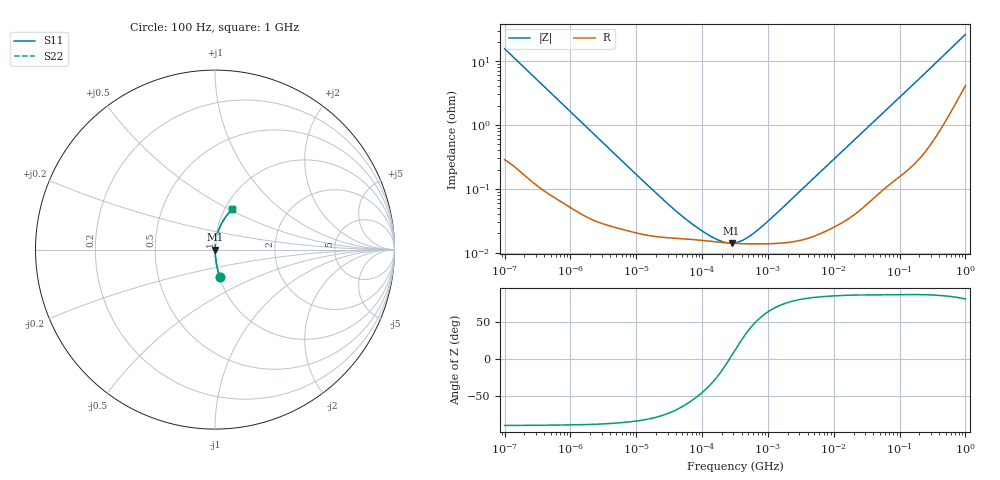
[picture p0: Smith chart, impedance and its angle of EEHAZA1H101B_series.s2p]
!  *** S-Parameter ***
!  Copyright (C) Panasonic Industry
!  Conductive Polymer Hybrid Aluminum Electrolytic Capacitor
!  Parts No. EEHAZA1H101B
!  Connection Mode : Series
!  1  o---||---o  2
!  GND o--------o GND
!  Conditions : Temperature = 20 degC , DC Bias = 0 V
! Frequency Range : 100Hz  -  1GHz  [ 401 Steps ]
# Hz S RI R 50
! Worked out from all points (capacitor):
!   401 points, 100 Hz to 1 GHz, reference 50 ohm
!   read as one part in series: C = 102 uF near 108.4 Hz
!   lowest |Z| = 14.1 mohm at 280.2 kHz (marker M1)
!   series resonance near 259.9 kHz, so ESL is about 3.7 nH
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100  0.0263 -0.151  0.9737 0.151  0.9737 0.151  0.0263 -0.151
108.3927  0.0228 -0.14  0.9772 0.14  0.9772 0.14  0.0228 -0.14
175.7924  0.00968 -0.0882  0.9903 0.0882  0.9903 0.0882  0.00968 -0.0882
309.0295  0.00372 -0.0509  0.9963 0.0509  0.9963 0.0509  0.00372 -0.0509
1487.647  0.000515 -0.0108  0.9995 0.0108  0.9995 0.0108  0.000515 -0.0108
22130.95  0.000177 -0.000758  0.9998 0.000758  0.9998 0.000758  0.000177 -0.000758
51582.22  0.000165 -0.000323  0.9998 0.000323  0.9998 0.000323  0.000165 -0.000323
102329.3  0.000155 -0.00015  0.9998 0.00015  0.9998 0.00015  0.000155 -0.00015
179887.1  0.000146 -5.53e-05  0.9999 5.53e-05  0.9999 5.53e-05  0.000146 -5.53e-05
229086.8  0.000143 -1.89e-05  0.9999 1.89e-05  0.9999 1.89e-05  0.000143 -1.89e-05
280220.6  0.000141 1.14e-05  0.9999 -1.14e-05  0.9999 -1.14e-05  0.000141 1.14e-05
316227.8  0.00014 3e-05  0.9999 -3e-05  0.9999 -3e-05  0.00014 3e-05
454464.5  0.000138 9.05e-05  0.9999 -9.05e-05  0.9999 -9.05e-05  0.000138 9.05e-05
707945.8  0.000137 0.000182  0.9999 -0.000182  0.9999 -0.000182  0.000137 0.000182
1295687  0.00014 0.000371  0.9999 -0.000371  0.9999 -0.000371  0.00014 0.000371
4704354  0.000179 0.00138  0.9998 -0.00138  0.9998 -0.00138  0.000179 0.00138
6.99842e7  0.00152 0.019  0.9985 -0.019  0.9985 -0.019  0.00152 0.019
1.566751e8  0.00399 0.0413  0.996 -0.0413  0.996 -0.0413  0.00399 0.0413
2.985383e8  0.011 0.0774  0.989 -0.0774  0.989 -0.0774  0.011 0.0774
5.922431e8  0.0376 0.1466  0.9624 -0.1466  0.9624 -0.1466  0.0376 0.1466
9.225714e8  0.0826 0.211  0.9174 -0.211  0.9174 -0.211  0.0826 0.211
1e9  0.0946 0.2237  0.9054 -0.2237  0.9054 -0.2237  0.0946 0.2237
